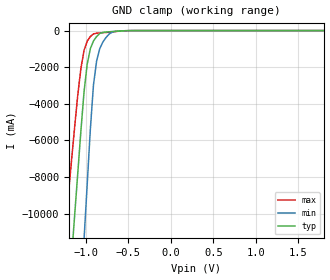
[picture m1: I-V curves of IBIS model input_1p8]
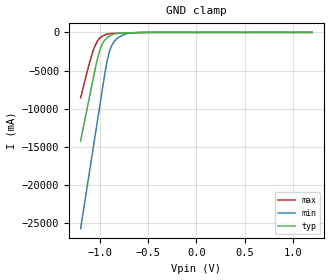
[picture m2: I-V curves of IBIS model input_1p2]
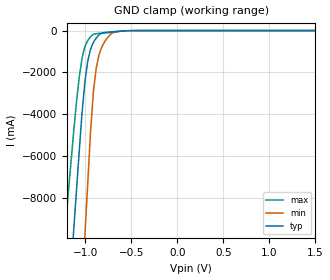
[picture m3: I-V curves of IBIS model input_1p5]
| IBIS file created by Layout Workbench Version 22.1.4.12161.401368   004
| Cadence Design Systems, Inc. 2011
[IBIS Ver]   4.2
[File name]   txb0604.ibs
[File Rev]  1.0
[Date]   16 05, 2026
[Source] Texas Instruments Incorporated.
[Notes]   - Added models for one-shot circuit for IO model
   - To generate the IO model for one-shot circuit, the one-shot paths are kept always active
   - Please note that models for one shot circuit on can be chosen under
   [Model Selector] for IO model.
   - Non-monotonic Pull-up behavior is expected
| TEXAS INSTRUMENTS INCORPORATED
| IBIS Model of TXB0604RUT,
| 4 bit Auto Bi-directional Voltage Level Translator
| This file contains package information for the following:
|  |  RUT 12-pin package
| The model is generated for 1.2V, 1.5V & 1.8V VCCA
| && 1.8V, 2.5V & 3.3V VCCB domains
| This file provides unique models under the [Model Selector] for each Vcc.
| For operation at a specific Vcc, select the appropriate model after each
| [Model Selector] keyword.
| Rev 1.0: 05/16/2026
| - Initial version of the model
| - Model generated from simulations in SPECTRE
| - C_comp although listed in numerical order of value are
|   obtained from varying PVT conditions. For PVT conditions for
|   each specific value refer the buffer description under
|   respective [Model]. IBIS model user is responsible for using
|   appropriate C_comp to simulate for Signal Integrity.
| - Warnings regarding combined Non-monotonicity of various models have been
|   reviewd and considered minor and can be ignored.
| - Model names with a trailing _2p25 contain the model for 2.25V operation.
|   Model names with a trailing _5p5 contain the model for 5.5V operation.
| This model is designed as an aid for customers of Texas Instruments.
| TI and its licensors and suppliers make no warranties, either expressed
| or implied, with respect to this  model, including the warranties of
| merchantability or fitness for a particular purpose. The model is
| provided solely on an "as is" basis. The entire risk as to its quality
| and performance is with the customer.
| This model is subject to change without notice. Texas Instruments
| Incorporated is not responsible for updating this model.
[Copyright]
 (C) Copyright 2026 Texas Instruments Incorporated.All rights reserved.
|   Component txb0604
[Component]   txb0604rut
[Manufacturer]   Texas Instruments, Inc.
[Package]   |UQFN, 16 pin RUT
| variable   typ   min   max
R_pkg   61.790m   31.580m   68.160m
L_pkg   0.635nH   0.412nH   0.783nH
C_pkg   0.223pF   0.172pF   0.269pF
[Pin]   signal_name   model_name   R_pin   L_pin   C_pin
1   VCCA   Power
2   A1   IO_LE
3   A2   IO_LE
4   A3   IO_LE
5   A4   IO_LE
6   GND   GND
7   B4   IO_RI
8   B3   IO_RI
9   B2   IO_RI
10   B1   IO_RI
11   VCCB   Power
12   OE   input
| Model input
[Model Selector]   input
input_1p2 	 1.2V VCCA
input_1p8 	 1.8V VCCA
input_1p5   1.5V VCCA
| Model IO_LE
[Model Selector]   IO_LE
IO_LE_1p2		 1.2V VCCA
IO_LE_1p5		 1.5V VCCA
IO_LE_1p8		 1.8V VCCA
IO_LE_OS_1p2	 1.2V VCCA -> One Shot path always ON
IO_LE_OS_1p5 	 1.5V VCCA -> One Shot path always ON
IO_LE_OS_1p8 	 1.8V VCCA -> One Shot path always ON
| Model IO_RI
[Model Selector]   IO_RI
IO_RI_1p8		 1.8V VCCB
IO_RI_2p5		 2.5V VCCB
IO_RI_3p3		 3.3V VCCB
IO_RI_OS_1p8	 1.8V VCCB -> One Shot path always ON
IO_RI_OS_2p5	 2.5V VCCB -> One Shot path always ON
IO_RI_OS_3p3 	 3.3V VCCB -> One Shot path always ON
| Models and submodels in the file (15): input_1p8 (Input), input_1p2 (Input), input_1p5 (Input), IO_LE_1p8 (3-state), IO_LE_1p2 (3-state), IO_LE_1p5 (3-state), IO_LE_OS_1p8 (3-state), IO_LE_OS_1p2 (3-state), IO_LE_OS_1p5 (3-state), IO_RI_1p8 (3-state), IO_RI_2p5 (3-state), IO_RI_3p3 (3-state), IO_RI_OS_1p8 (3-state), IO_RI_OS_2p5 (3-state), IO_RI_OS_3p3 (3-state)
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|   Model input_1p8
[Model] input_1p8
Model_type Input
Polarity   Non-Inverting
Enable   Active-High
Vinl =  0.630V
Vinh =  1.170V
C_comp   0.530pF   0.360pF   0.720pF
[Temperature Range]   27.000   0.125k   -40.000
[Voltage Range]   1.800V   1.650V   1.950V
[POWER Clamp Reference]   1.800V   1.650V   1.950V
[GND Clamp Reference]   0.0V   0.0V   0.0V
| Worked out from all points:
|   GND clamp passes 1 mA (typ) near -0.44 V on its own axis
[GND_clamp]
|Voltage   I(typ)   I(min)   I(max)
-1.8V     -51.89A    -74.38A    -38.5A
-1.245V   -17.07A    -29.39A    -10.81A
-1.171V   -12.43A    -23.39A    -7.12A
-1.134V   -10.11A    -20.39A    -5.274A
-1.06V    -5.465A    -14.4A     -2.06A
-1.023V   -3.334A    -11.4A     -1.077A
-986mV    -1.832A    -8.396A    -580.6mA
-912mV    -568.5mA   -2.968A    -181.7mA
-875mV    -324mA     -1.654A    -144mA
-838mV    -157.5mA   -986.7mA   -128.1mA
-690mV    -51.94mA   -86.18mA   -69.46mA
1.8V      0A         0A         0A
[Model] input_1p2
Model_type Input
Polarity   Non-Inverting
Enable   Active-High
Vinl =  0.420V
Vinh =  0.780V
C_comp   0.550pF   0.380pF   0.760pF
[Temperature Range]   27.000   0.125k   -40.000
[Voltage Range]   1.200V   1.100V   1.300V
[POWER Clamp Reference]   1.200V   1.100V   1.300V
[GND Clamp Reference]   0.0V   0.0V   0.0V
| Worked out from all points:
|   GND clamp passes 1 mA (typ) near -0.44 V on its own axis
[GND_clamp]
|Voltage   I(typ)   I(min)   I(max)
-1.2V     -14.25A    -25.74A    -8.567A
-1.075V   -6.406A    -15.61A    -2.602A
-1.025V   -3.434A    -11.56A    -1.116A
-1V       -2.317A    -9.531A    -724.2mA
-975mV    -1.518A    -7.504A    -491.3mA
-925mV    -686mA     -3.674A    -213.4mA
-900mV    -478.3mA   -2.444A    -164.1mA
-875mV    -324mA     -1.655A    -144mA
-825mV    -130mA     -835.6mA   -123.8mA
-725mV    -65.57mA   -176.2mA   -87.04mA
-625mV    -28.76mA   -30.2mA    -38.19mA
1.2V      0A         0A         0A
[Model] input_1p5
Model_type Input
Polarity   Non-Inverting
Enable   Active-High
Vinl =  0.600V
Vinh =  1.000V
C_comp   0.540pF   0.360pF   0.740pF
[Temperature Range]   27.000   0.125k   -40.000
[Voltage Range]   1.500V   1.400V   1.600V
[POWER Clamp Reference]   1.500V   1.400V   1.600V
[GND Clamp Reference]   0.0V   0.0V   0.0V
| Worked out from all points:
|   GND clamp passes 1 mA (typ) near -0.44 V on its own axis
[GND_clamp]
|Voltage   I(typ)   I(min)   I(max)
-1.5V     -33.07A    -50.06A    -23.54A
-1.221V   -15.57A    -27.45A    -9.614A
-1.128V   -9.731A    -19.91A    -4.974A
-1.066V   -5.841A    -14.88A    -2.269A
-1.004V   -2.476A    -9.855A    -774.3mA
-973mV    -1.469A    -7.342A    -476.7mA
-942mV    -884.9mA   -4.837A    -289.9mA
-911mV    -560.5mA   -2.921A    -179.9mA
-880mV    -352.3mA   -1.785A    -147mA
-818mV    -119.5mA   -765.6mA   -121.5mA
-663mV    -41.74mA   -53.83mA   -55.81mA
1.5V      0A         0A         0A
